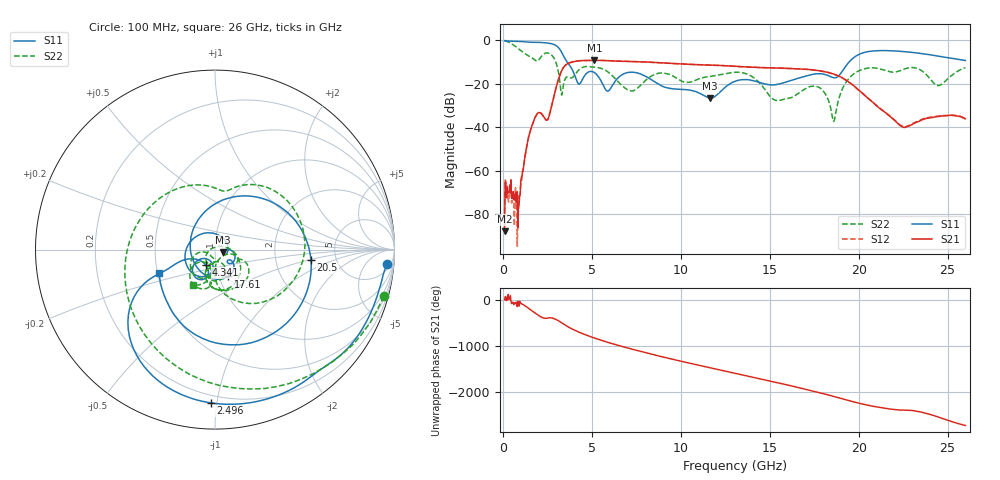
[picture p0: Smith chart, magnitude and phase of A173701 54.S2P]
!  2-Port S-parameters saved by WinCal
! VAR MeasName=S-Parameters (CALIBRATED_DATA) read from VNA (N5245A)
! VAR MeasDate=2017-6-7 10:31:59
! VAR NAME=A173701 54
! VAR FILENAME=A173701 54.S2P
! VAR DATE=2017-6-7 10:31:59
! VAR PHYS_PORTS=1,2
# Hz S DB R 50
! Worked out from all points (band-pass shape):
!   801 points, 100 MHz to 26 GHz, reference 50 ohm
!   highest |S21| = -9.35 dB at 5.151 GHz (marker M1); lowest = -88.0 dB at 100 MHz (marker M2)
!   |S21| within 3 dB of the highest: 3.433 GHz to 13.6 GHz (10.17 GHz wide, 119 % of centre); 13.61324 GHz to 13.64526 GHz (32.02 MHz wide, 0.235 % of centre)
!   lowest |S11| = -26.8 dB at 11.66 GHz (marker M3), VSWR 1.10, Z = 54.5 - j1.6 ohm
!   |S11| at or under -10 dB: 3.606 GHz to 19.48 GHz (15.87 GHz wide, 138 % of centre)
!   |S22| runs from -37.4 to -0.2 dB; largest |S21 - S12| = 0.0035
!   S11 on the Smith chart (normalised r, x): 100 MHz: 9, -20; 2.496 GHz: 0.15, -0.96; 4.341 GHz: 0.89, -0.15; 17.61 GHz: 1.11, -0.34; 20.5 GHz: 3.23, -0.54; 26 GHz: 0.51, -0.15
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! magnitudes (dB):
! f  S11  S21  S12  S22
! 100 MHz  -0.3  -88.0  -79.5  -0.2
! 877 MHz  -0.6  -77.7  -71.7  -4.0
! 1.686 GHz  -1.0  -38.3  -38.2  -8.5
! 2.496 GHz  -1.4  -36.8  -36.8  -6.0
! 3.337 GHz  -6.1  -13.6  -13.6  -24.4
! 4.341 GHz  -20.0  -9.5  -9.5  -13.2
! 4.438 GHz  -18.7  -9.5  -9.5  -12.7
! 5.151 GHz  -15.0  -9.4  -9.4  -12.5
! 5.895 GHz  -23.5  -9.5  -9.5  -14.6
! 7.19 GHz  -14.8  -9.9  -9.8  -23.4
! 8.744 GHz  -20.3  -10.4  -10.4  -15.3
! 11.66 GHz  -26.8  -11.5  -11.5  -16.7
! 13.05 GHz  -19.0  -12.1  -12.1  -14.8
! 15.38 GHz  -20.5  -12.9  -12.9  -27.7
! 17.39 GHz  -15.8  -13.8  -13.7  -21.3
! 17.61 GHz  -15.5  -13.9  -13.9  -21.3
! 18.62 GHz  -17.4  -15.7  -15.7  -37.2
! 19.3 GHz  -11.8  -18.5  -18.5  -19.3
! 20.5 GHz  -5.4  -26.6  -26.6  -12.9
! 21.69 GHz  -4.9  -34.7  -34.5  -14.5
! 24.48 GHz  -7.4  -35.1  -34.9  -21.0
! 26 GHz  -9.4  -36.2  -36.3  -12.7
